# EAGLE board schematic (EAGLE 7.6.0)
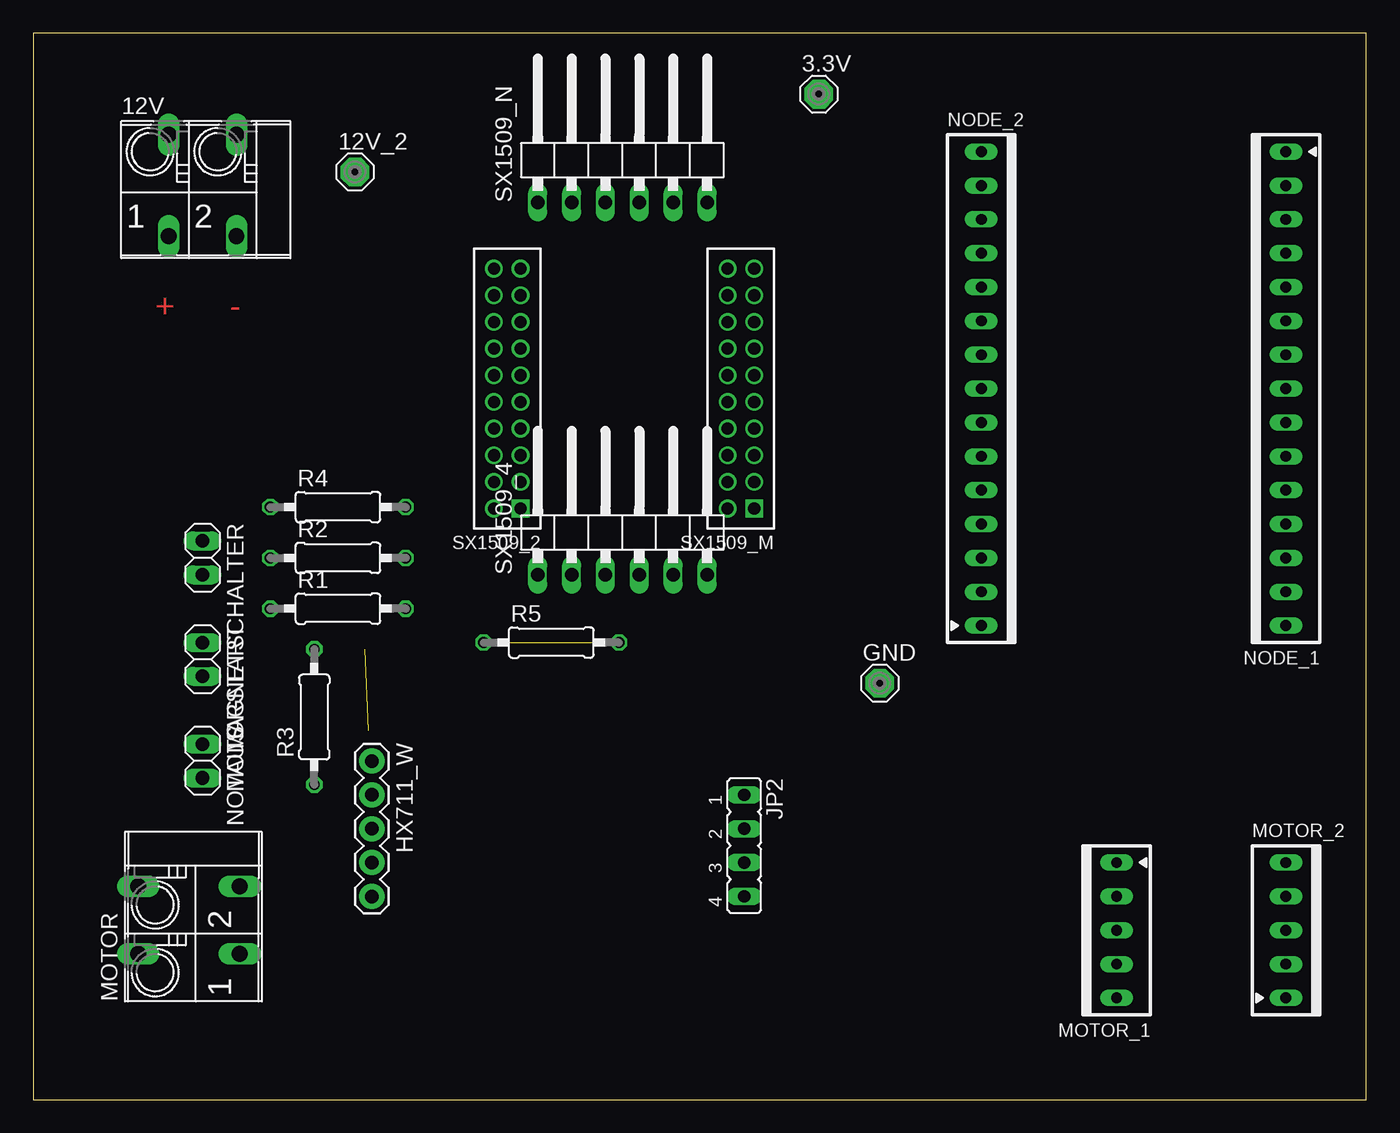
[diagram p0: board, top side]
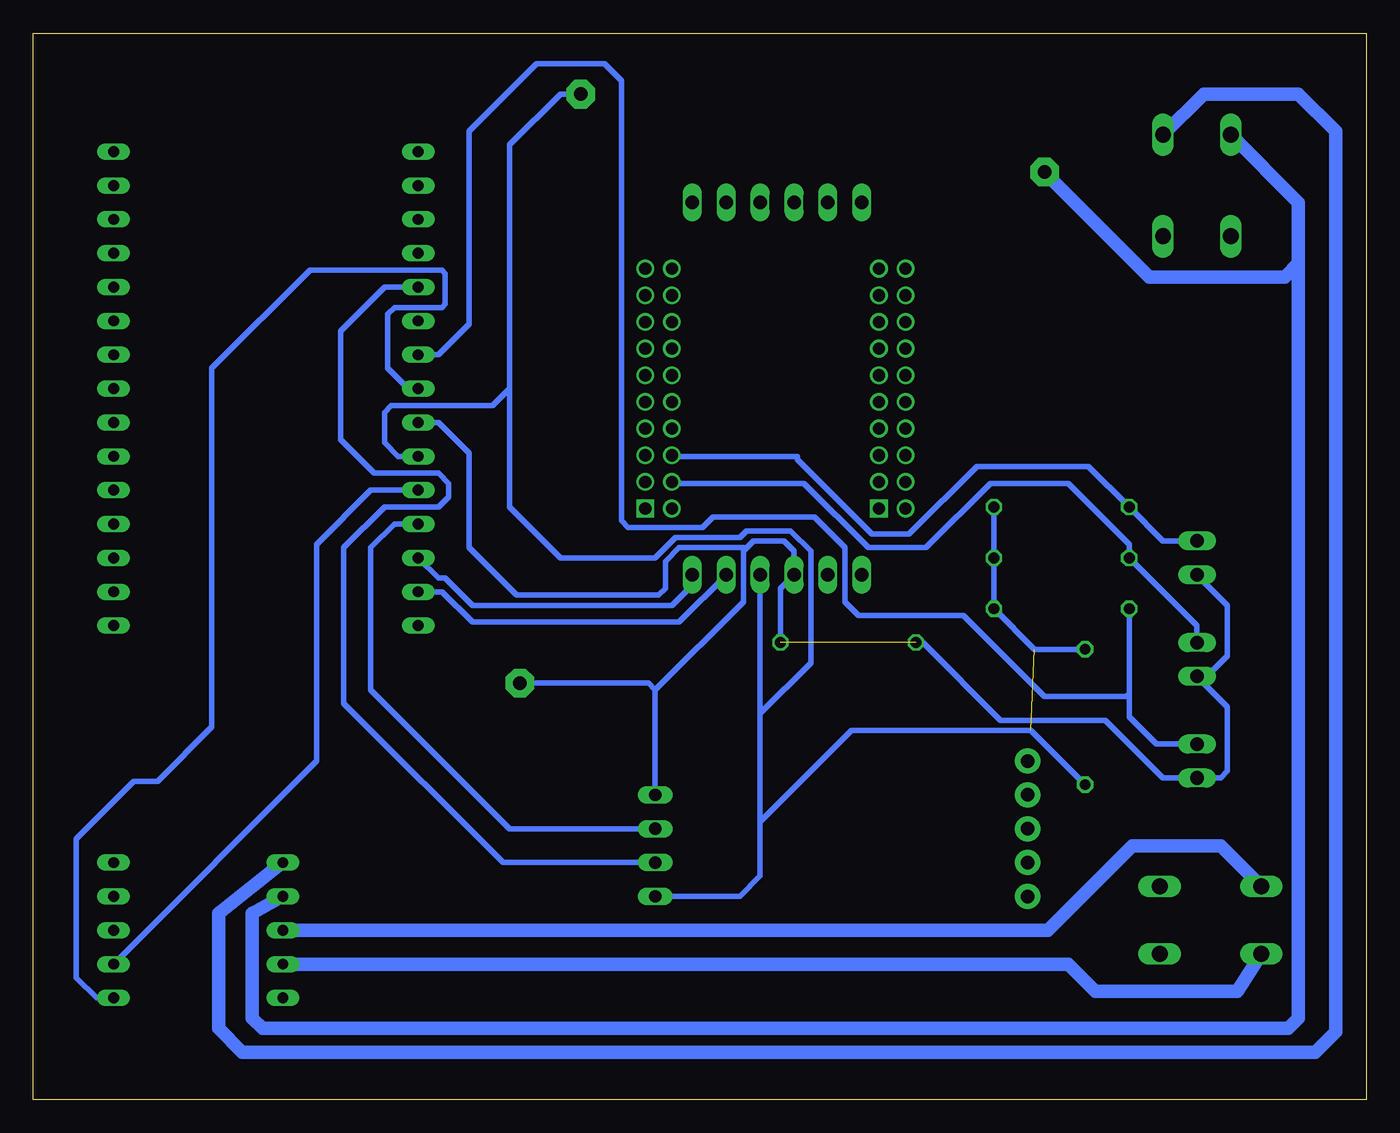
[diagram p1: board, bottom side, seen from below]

Size 100 x 80 mm. Coordinates in mm from the lower left corner, seen from the top.
Outline: 0,0 100,0 100,80 0,80 0,0
Copper layers (1*16): Top 0.035mm / dielectric 1.5mm / Bottom 0.035mm
Design rules "PCB-POOL": minimum track width 6mil, minimum drill 12mil, track to track 6mil, track to pad 6mil, pad to pad 6mil, via to via 6mil, smd to smd 6mil, copper to edge 20mil, drill to drill 8mil, minimum pad ring 8mil, minimum via ring 6mil, stop-mask expansion 3mil, vias tented up to drill 0mil, thermal gap 8mil

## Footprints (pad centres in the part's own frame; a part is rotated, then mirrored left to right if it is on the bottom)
MCS10B = drill 1.016 pad 2.159 octagon: MP 0,0
FFKV2 = drill 1.194 long: 1 -2.54,-3.81; 1A -2.54,3.81; 2 2.54,-3.81; 2A 2.54,3.81
1X05 = drill 1.016 pad 1.88: 1 0,0; 2 2.54,0; 3 5.08,0; 4 7.62,0; 5 10.16,0
JP4 = drill 0.914 long: 1 -3.81,0; 2 -1.27,0; 3 1.27,0; 4 3.81,0
1X02 = drill 1.016 long: 1 -1.27,0; 2 1.27,0
LCW-105-XX-X-S = drill 0.813 long: 1 5.08,0; 2 2.54,0; 3 0,0; 4 -2.54,0; 5 -5.08,0
LCW-115-XX-X-S = drill 0.813 long: 1 17.78,0; 2 15.24,0; 3 12.7,0; 4 10.16,0; 5 7.62,0; 6 5.08,0; 7 2.54,0; 8 0,0; 9 -2.54,0; 10 -5.08,0; 11 -7.62,0; 12 -10.16,0; 13 -12.7,0; 14 -15.24,0; 15 -17.78,0
0207/10 = drill 0.813 octagon: 1 -5.08,0; 2 5.08,0
87758-20 = drill 0.914 square: 1 -9,-1 | drill 0.914: 2 -9,1; 3 -7,-1; 4 -7,1; 5 -5,-1; 6 -5,1; 7 -3,-1; 8 -3,1; 9 -1,-1; 10 -1,1; 11 1,-1; 12 1,1; 13 3,-1; 14 3,1; 15 5,-1; 16 5,1; 17 7,-1; 18 7,1; 19 9,-1; 20 9,1
1X06/90 = drill 1.016 long: 1 -6.35,-3.81; 2 -3.81,-3.81; 3 -1.27,-3.81; 4 1.27,-3.81; 5 3.81,-3.81; 6 6.35,-3.81

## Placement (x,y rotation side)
3.3V  MCS10B  [MCS10B]  58.93,75.44 0 top
12V  FFKV2  [FFKV2]  12.7,68.58 0 top
12V_2  MCS10B  [MCS10B]  24.13,69.6 0 top
GND  MCS10B  [MCS10B]  63.5,31.24 0 top
HX711_W  [1X05]  25.4,25.4 270 top
JP2  [JP4]  53.34,19.05 270 top
MAGNETSCHALTER  [1X02]  12.7,40.64 270 top
MOTOR  FFKV2  [FFKV2]  11.68,13.46 90 top
MOTOR_1  LCW-105-XX-X-S  [LCW-105-XX-X-S]  81.28,12.7 90 top
MOTOR_2  LCW-105-XX-X-S  [LCW-105-XX-X-S]  93.98,12.7 270 top
MOTORSTART  [1X02]  12.7,33.02 270 top
NODE_1  LCW-115-XX-X-S  [LCW-115-XX-X-S]  93.98,53.34 90 top
NODE_2  LCW-115-XX-X-S  [LCW-115-XX-X-S]  71.12,53.34 270 top
NOTAUS  [1X02]  12.7,25.4 270 top
R1  10k  [0207/10]  22.86,36.83 0 top
R2  10k  [0207/10]  22.86,40.64 0 top
R3  0  [0207/10]  21.08,28.7 90 top
R4  10k  [0207/10]  22.86,44.45 0 top
R5  0  [0207/10]  38.86,34.29 0 top
SX1509_2  87758-20  [87758-20]  35.56,53.34 90 top
SX1509_4  [1X06/90]  44.2,43.18 0 top
SX1509_M  87758-20  [87758-20]  53.09,53.34 90 top
SX1509_N  [1X06/90]  44.2,71.12 0 top

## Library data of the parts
3.3V 12V_2 GND = solpad
12V MOTOR = con-phoenix-508; OC_FARNELL: unknown; OC_NEWARK: unknown
HX711_W = SparkFun-Connectors
JP2 = jumper
MAGNETSCHALTER MOTORSTART NOTAUS SX1509_4 SX1509_N = pinhead
MOTOR_1 MOTOR_2 NODE_1 NODE_2 = con-samtec
R1-R5 = eagle-ltspice; SPICEMODEL: NONE; SPICEPREFIX: R
SX1509_2 SX1509_M = con-molex-milli-grid

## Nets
GND: GND.MP JP2.1 MAGNETSCHALTER.2 MOTORSTART.2 NODE_2.7 NOTAUS.2 R5.1 R5.2 SX1509_4.3
N$1: NODE_2.2 SX1509_4.5
N$2: NODE_2.3 SX1509_4.6
N$3: MOTOR_2.1 NODE_2.8
N$4: MOTOR_2.2 NODE_2.5
N$5: JP2.2 NODE_2.4
N$6: JP2.3 NODE_2.11
N$7: 12V.2A MOTOR_1.1
N$8: 12V.1A 12V_2.MP MOTOR_1.2
N$9: MOTOR.2A MOTOR_1.3
N$10: MOTOR.1A MOTOR_1.4
N$11: MOTORSTART.1 R2.1 SX1509_M.4
N$14: NODE_2.9 NOTAUS.1 R1.1
N$16: MAGNETSCHALTER.1 R4.1 SX1509_M.6
VCC: 3.3V.MP JP2.4 NODE_2.6 R1.2 R2.2 R3.1 R3.2 R4.2 SX1509_4.4

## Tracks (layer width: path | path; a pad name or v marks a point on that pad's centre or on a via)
GND  (1 unrouted)
  Bottom 0.406: JP2.1 53.34,30.73 | 53.34,30.73 46.74,37.34 46.74,41.15 46.61,41.27 | 46.61,41.27 45.97,41.91 43.69,41.91 42.93,41.15 SX1509_4.3 43.94,38.35 R5.2 | GND.MP 53.85,31.24 53.34,30.73 | R5.1 33.27,34.29 27.43,28.45 19.56,28.45 15.24,24.13 NOTAUS.2 10.92,24.13 10.41,24.64 10.41,29.46 MOTORSTART.2 11.94,31.75 10.41,33.27 10.41,37.08 MAGNETSCHALTER.2 | NODE_2.7 69.6,50.8 67.31,48.51 67.31,41.4 63.75,37.85 53.09,37.85 52.58,38.35 52.58,40.39 51.56,41.4 46.74,41.4 46.61,41.27
N$1
  Bottom 0.406: NODE_2.2 69.34,38.1 67.06,35.81 51.56,35.81 SX1509_4.5
N$2
  Bottom 0.406: SX1509_4.6 50.55,38.61 52.07,37.08 67.06,37.08 69.09,39.12 69.6,39.12 NODE_2.3
N$3
  Bottom 0.406: MOTOR_2.1 95.25,7.62 96.77,9.14 96.77,19.56 92.46,23.88 90.68,23.88 86.61,27.94 86.61,54.86 79.25,62.23 69.34,62.23 69.09,61.98 69.09,59.69 69.34,59.44 72.9,59.44 73.41,58.93 73.41,54.86 71.88,53.34 NODE_2.8
N$4
  Bottom 0.406: NODE_2.5 74.68,45.72 78.74,41.66 78.74,25.4 MOTOR_2.2
N$5
  Bottom 0.406: NODE_2.4 72.9,43.18 74.68,41.4 74.68,30.73 64.26,20.32 JP2.2
N$6
  Bottom 0.406: NODE_2.11 73.66,60.96 76.96,57.66 76.96,49.53 74.42,46.99 69.6,46.99 68.83,46.23 68.83,45.21 69.6,44.45 73.66,44.45 76.71,41.4 76.71,29.72 64.77,17.78 JP2.3
N$7
  Bottom 1.016: MOTOR_1.1 86.11,13.97 86.11,5.33 84.33,3.56 3.81,3.56 2.29,5.08 2.29,72.64 5.08,75.44 12.19,75.44 12V.2A
N$8
  Bottom 1.016: MOTOR_1.2 83.57,13.97 83.57,6.1 82.8,5.33 5.84,5.33 5.08,6.1 5.08,62.74 | 12V_2.MP 16.26,61.72 6.1,61.72 5.08,62.74 | 5.08,62.74 5.08,67.31 12V.1A
N$9
  Bottom 1.016: MOTOR_1.3 23.88,12.7 17.53,19.05 10.92,19.05 MOTOR.2A
N$10
  Bottom 1.016: MOTOR_1.4 22.35,10.16 20.32,8.13 9.65,8.13 MOTOR.1A
N$11
  Bottom 0.406: MOTORSTART.1 12.7,35.56 R2.1 17.78,41.66 22.35,46.23 28.19,46.23 33.02,41.4 37.34,41.4 42.16,46.23 51.97,46.23 SX1509_M.4
N$14
  Bottom 0.406: 17.78,30.48 17.78,28.7 15.75,26.67 NOTAUS.1 | 17.78,30.48 R1.1 | NODE_2.9 69.6,55.88 67.31,58.17 67.31,72.64 62.23,77.72 57.15,77.72 55.88,76.45 55.88,43.43 55.37,42.93 49.78,42.93 49.02,43.69 41.4,43.69 39.12,41.4 39.12,37.34 38.1,36.32 30.23,36.32 24.13,30.23 18.03,30.23 17.78,30.48
N$16
  Bottom 0.406: MAGNETSCHALTER.1 15.24,41.91 R4.1 20.83,47.5 29.21,47.5 34.29,42.42 37.08,42.42 42.67,48.01 42.67,48.26 52.01,48.26 SX1509_M.6
VCC  (1 unrouted)
  Bottom 0.406: JP2.4 46.99,15.24 45.47,16.76 45.47,20.83 | SX1509_4.4 45.47,28.96 | 45.47,28.96 45.47,20.83 | 64.26,53.34 64.26,44.45 60.45,40.64 53.34,40.64 51.82,42.16 46.99,42.16 46.48,42.67 43.18,42.67 41.66,41.15 41.66,32.77 45.47,28.96 | 64.26,53.34 64.26,71.63 60.45,75.44 3.3V.MP | 45.47,20.83 38.61,27.69 25.15,27.69 R3.1 | R4.2 R2.2 R1.2 24.89,33.78 R3.2 | NODE_2.6 72.64,48.26 73.66,49.28 73.66,51.56 73.15,52.07 65.53,52.07 64.26,53.34

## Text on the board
Top: + | -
